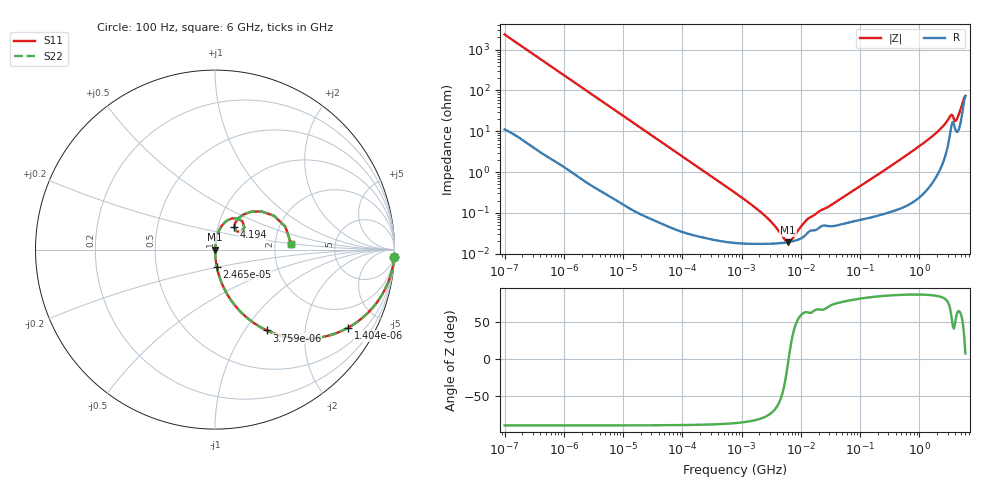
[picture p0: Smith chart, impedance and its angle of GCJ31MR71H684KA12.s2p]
!Murata Part Number: GCJ31MR71H684KA12
!These Parameters are Measured in Series Mode Connection
!Data Generated on Mar 13, 2026
!  o--ll--o
!Port1  Port2
!  o------o
!Operation Temp=25[degC], DC Bias Voltage=0[V]
!Freq. Start=100[Hz] Stop=6[GHz] 401[Steps]
# Hz S RI R 50
!Freq.(Hz) S11(Real) S11(Imag) S21(Real) S21(Imag) S12(Real) S12(Imag) S22(Real) S22(Imag)
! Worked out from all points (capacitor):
!   401 points, 100 Hz to 6 GHz, reference 50 ohm
!   read as one part in series: C = 674 nF near 109 Hz
!   lowest |Z| = 19.1 mohm at 6.075 MHz (marker M1)
!   series resonance near 6.228 MHz, so ESL is about 970 pH
!   S11 on the Smith chart (normalised r, x): 100 Hz: 1, -47; 1.404 kHz: 1.02, -3.39; 3.759 kHz: 1.01, -1.27; 24.65 kHz: 1.00, -0.20; 4.194 GHz: 1.20, +0.31; 6 GHz: 2.46, +0.19
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100  0.998 -0.0423  0.00199 0.0423  0.00199 0.0423  0.998 -0.0423
548  0.9482 -0.2189  0.0518 0.2189  0.0518 0.2189  0.9482 -0.2189
1404  0.7407 -0.4355  0.2593 0.4355  0.2593 0.4355  0.7407 -0.4355
2008  0.5842 -0.4901  0.4158 0.4901  0.4158 0.4901  0.5842 -0.4901
3759  0.2886 -0.4502  0.7114 0.4502  0.7114 0.4502  0.2886 -0.4502
8047  0.0828 -0.2724  0.9172 0.2724  0.9172 0.2724  0.0828 -0.2724
24648  0.0102 -0.0965  0.9898 0.0965  0.9898 0.0965  0.0102 -0.0965
40335  0.00413 -0.0594  0.9959 0.0594  0.9959 0.0594  0.00413 -0.0594
774597  0.000192 -0.00311  0.9998 0.00311  0.9998 0.00311  0.000192 -0.00311
2594782  0.000174 -0.000779  0.9998 0.000779  0.9998 0.000779  0.000174 -0.000779
5311619  0.000185 -0.000126  0.9998 0.000126  0.9998 0.000126  0.000185 -0.000126
6075234  0.00019 -1.94e-05  0.9998 1.94e-05  0.9998 1.94e-05  0.00019 -1.94e-05
6948629  0.000197 8.67e-05  0.9998 -8.67e-05  0.9998 -8.67e-05  0.000197 8.67e-05
1.189169e7  0.00028 0.000549  0.9997 -0.000549  0.9997 -0.000549  0.00028 0.000549
1.555665e7  0.000371 0.000731  0.9996 -0.000731  0.9996 -0.000731  0.000371 0.000731
3.124326e8  0.0012 0.0133  0.9988 -0.0133  0.9988 -0.0133  0.0012 0.0133
1.565993e9  0.00962 0.0694  0.9904 -0.0694  0.9904 -0.0694  0.00962 0.0694
2.562649e9  0.0351 0.1285  0.9649 -0.1285  0.9649 -0.1285  0.0351 0.1285
3.205649e9  0.0953 0.1739  0.9047 -0.1739  0.9047 -0.1739  0.0953 0.1739
4.193612e9  0.1078 0.1255  0.8922 -0.1255  0.8922 -0.1255  0.1078 0.1255
5.016141e9  0.2032 0.2113  0.7968 -0.2113  0.7968 -0.2113  0.2032 0.2113
6e9  0.4241 0.0317  0.5759 -0.0317  0.5759 -0.0317  0.4241 0.0317
